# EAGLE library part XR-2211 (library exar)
FSK demodulator TONE DECODER
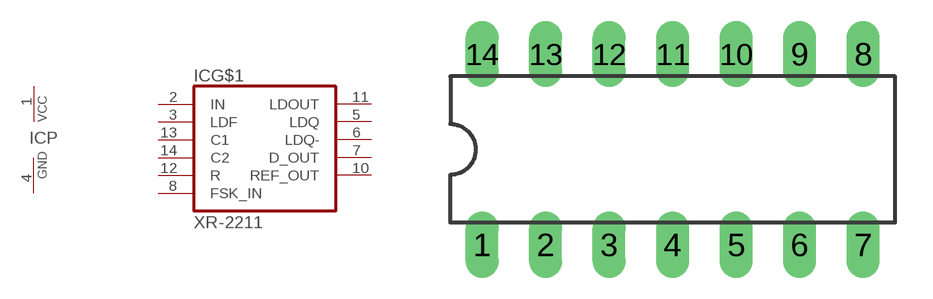
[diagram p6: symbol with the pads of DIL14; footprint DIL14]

Designator prefix IC; gates G$1=XR-2211 P=PWRN

## XR-2211 (OC_FARNELL: unknown; OC_NEWARK: unknown)  [DIL14]
1  P:VCC  pwr
2  G$1:IN  in
3  G$1:LDF  in
4  P:GND  pwr
5  G$1:LDQ  out
6  G$1:LDQ-  out
7  G$1:D_OUT  out
8  G$1:FSK_IN  in
10  G$1:REF_OUT  out
11  G$1:LDOUT  out
12  G$1:R  in
13  G$1:C1  in
14  G$1:C2  in

## Footprint DIL14 (pad centres in mm)
Dual In Line Package
drill 0.813 long: 1 -7.62,-3.81; 2 -5.08,-3.81; 3 -2.54,-3.81; 4 0,-3.81; 5 2.54,-3.81; 6 5.08,-3.81; 7 7.62,-3.81; 8 7.62,3.81; 9 5.08,3.81; 10 2.54,3.81; 11 0,3.81; 12 -2.54,3.81; 13 -5.08,3.81; 14 -7.62,3.81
